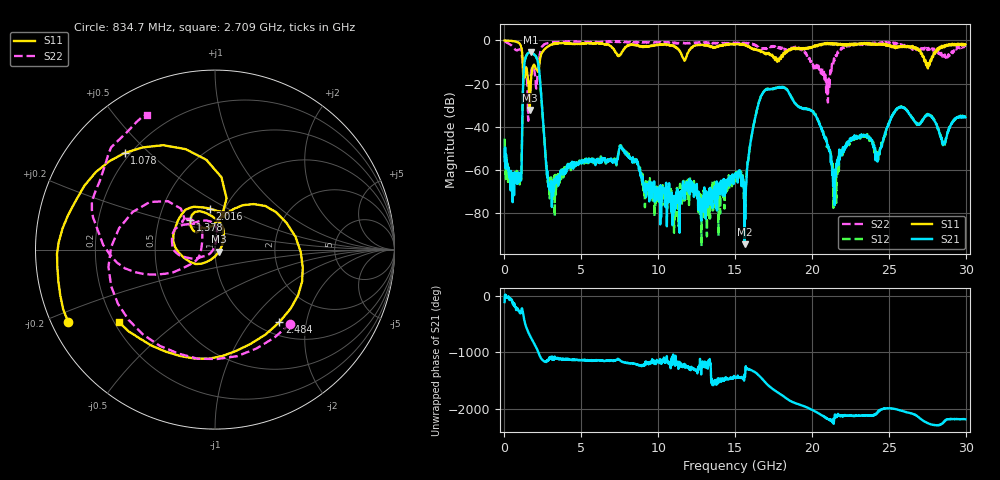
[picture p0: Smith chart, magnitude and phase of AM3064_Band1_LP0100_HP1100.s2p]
# Hz S DB R 50.0
!freq dBS11 angS11 dBS21 angS21 dBS12 angS12 dBS22 angS22
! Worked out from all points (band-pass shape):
!   1600 points, 10 MHz to 29.98 GHz, reference 50 ohm
!   highest |S21| = -5.57 dB at 1.697 GHz (marker M1); lowest = -94.3 dB at 15.62 GHz (marker M2)
!   |S21| within 3 dB of the highest: 1.352 GHz to 2.114 GHz (762.6 MHz wide, 44 % of centre)
!   lowest |S11| = -32.2 dB at 1.641 GHz (marker M3), VSWR 1.05, Z = 52.2 - j1.15 ohm
!   |S11| at or under -10 dB: 1.186 GHz to 2.29 GHz (1.103 GHz wide, 63.5 % of centre); 27.4 GHz to 27.68 GHz (281.3 MHz wide, 1.02 % of centre)
!   |S22| runs from -37.2 to -0.4 dB; largest |S21 - S12| = 0.008
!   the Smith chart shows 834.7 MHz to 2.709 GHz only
!   S11 on the Smith chart (normalised r, x): 834.7 MHz: 0.05, -0.23; 1.078 GHz: 0.18, +0.42; 1.378 GHz: 0.72, +0.25; 2.016 GHz: 0.85, +0.41; 2.484 GHz: 1.23, -1.41; 2.709 GHz: 0.22, -0.32
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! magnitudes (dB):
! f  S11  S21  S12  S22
! 10 MHz  0.0  -50.1  -45.5  -0.4
! 834.7 MHz  -0.8  -63.0  -62.8  -4.6
! 1.078 GHz  -2.6  -64.9  -64.5  -4.8
! 1.378 GHz  -13.4  -7.9  -7.9  -14.5
! 1.641 GHz  -32.2  -5.6  -5.5  -20.1
! 1.697 GHz  -21.3  -5.6  -5.5  -16.8
! 2.016 GHz  -12.7  -7.1  -7.1  -18.0
! 2.484 GHz  -5.3  -34.4  -34.4  -2.6
! 2.709 GHz  -3.5  -56.1  -57.9  -1.5
! 3.009 GHz  -2.1  -66.1  -67.0  -1.0
! 5.015 GHz  -1.4  -55.4  -56.3  -0.7
! 7.639 GHz  -5.4  -50.1  -50.0  -0.7
! 10 GHz  -2.0  -69.8  -73.3  -1.0
! 15 GHz  -1.8  -61.9  -62.4  -1.4
! 15.62 GHz  -2.0  -94.3  -72.4  -1.1
! 16.9 GHz  -6.1  -23.4  -23.4  -3.9
! 19.99 GHz  -3.5  -32.7  -32.5  -11.0
! 21.02 GHz  -1.2  -48.4  -49.3  -26.6
! 21.51 GHz  -1.4  -61.1  -63.5  -8.7
! 25 GHz  -2.0  -39.0  -38.3  -1.2
! 28.58 GHz  -2.9  -47.7  -47.7  -7.4
! 29.98 GHz  -1.8  -35.6  -35.4  -3.0
